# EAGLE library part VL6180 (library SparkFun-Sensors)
ST VL6180X Proximity and Ambient Light Sensing (ALS) Module Instead of estimating the distance by measuring the amount of light reflected back from the object (which is significantly influenced by color and surface), the VL6180 precisely measures the time the light takes to travel to the nearest object and reflect back to the sensor (Time-of-Flight). Combining an IR emitter, a range sensor and an ambient light sensor in a three-in-one ready-to-use reflowable package, the VL6180 is easy to integrate and saves the end-product makers the long and costly optical and mechanical design optimizations. Datasheet SparkFun Products SparkFun ToF Range Finder Breakout - VL6180 (SEN-12784) SparkFun ToF Range Finder Sensor - VL6180 (SEN-12785)
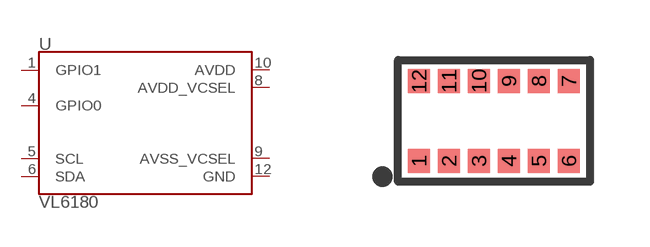
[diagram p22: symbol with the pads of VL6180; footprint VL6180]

Designator prefix U

## VL6180 (PROD_ID: IC-12007)  [VL6180]
1  GPIO1
4  GPIO0
5  SCL
6  SDA
8  AVDD_VCSEL
9  AVSS_VCSEL
10  AVDD
12  GND

## Footprint VL6180 (pad centres in mm)
VL6180 Specifications: Pin Count: 12 Area: 4.8 x 2.8 mm Pitch: 0.75mm Devices Using: VL6180
smd 0.55 x 0.6: 1 -1.875,-1; 2 -1.125,-1; 3 -0.375,-1; 4 0.375,-1; 5 1.125,-1; 6 1.875,-1; 7 1.875,1; 8 1.125,1; 9 0.375,1; 10 -0.375,1; 11 -1.125,1; 12 -1.875,1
